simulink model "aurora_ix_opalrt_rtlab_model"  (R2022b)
settings: Solver=ode3  StartTime=0.0  StopTime=inf  FixedStep=Ts  RelTol=1e-3
PostLoadFcn:
  | aurora_ix_opalrt_rtlab_param;
InitFcn:
  | aurora_ix_opalrt_rtlab_param;
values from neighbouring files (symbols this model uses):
  Ts = 20e-6    (= 2e-05)    [aurora_ix_opalrt_rtlab_param.m]
undefined symbols (not defined in the file or in its folder): af15, arm1_g1, aurora_ix_opalrt_rtlab, aurora_ix_opalrt_rtlab_ehs, aurora_ix_opalrt_rtlab_model, aurora_ix_opalrt_rtlab_param, Boost2lvl_SFun, boost_I, boost_V, C, c62c8459, DB, EFPGASIMConfig, eHSBuildReport, eHSx64_Gen4_Machines_IOConfig1, EX, fault_sw, LABv2024, logs, matlab, Min, models, ns, OPAL, RT, Step, TE0741_3, Time, Users, v1, vin, vsrc1, vsrc2, vsrc3
libraries: rtlab x5, opal_lib x3, rtio_opalrt_common x3, monitoringUserLib x1, ehsSchematicEditorSourceLib x1

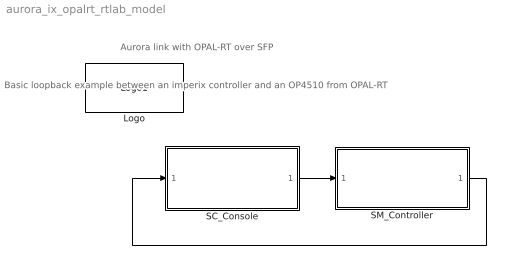
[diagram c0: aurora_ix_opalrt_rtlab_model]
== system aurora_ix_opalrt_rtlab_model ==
  note: Aurora link with OPAL-RT over SFP
  note: Basic loopback example between an imperix controller and an OP4510 from OPAL-RT
  Logo : opal_lib/Logo1  vide=[]
  SC_Console : Subsystem
  SM_Controller : Subsystem
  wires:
  SC_Console/1(to_eHS) -> SM_Controller/1(to_eHS)
  SM_Controller/1(from_eHS) -> SC_Console/1(from_eHS)

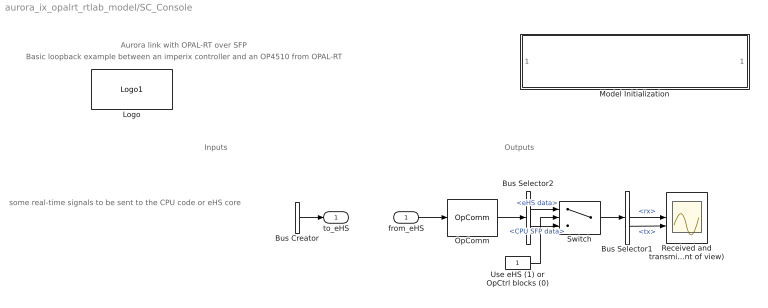
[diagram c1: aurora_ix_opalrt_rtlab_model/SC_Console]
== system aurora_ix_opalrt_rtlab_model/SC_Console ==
  note: some real-time signals to be sent to the CPU code or eHS core
  note: Inputs
  note: Outputs
  note: Aurora link with OPAL-RT over SFP
  note: Basic loopback example between an imperix controller and an OP4510 from OPAL-RT
  from_eHS : Inport  OutDataTypeStr=double
  Bus Creator : BusCreator  Inputs=2
  Bus Selector1 : BusSelector  OutputSignals=rx,tx
  Bus Selector2 : BusSelector  OutputSignals=eHS data,CPU SFP data
  Logo : opal_lib/Logo1  vide=[]
  Model Initialization : Subsystem  mask(Model Functions){InitFcnX=aurora_ix_opalrt_rtlab_param;, prel=off, posl=on, inif=on, strf=off}
      mask prompts: InitFcnX "Initialisation"; prel "Preload Function"; posl "PostLoad Function"; inif "InitFcn"; strf "StartFcn"
      mask init:
      | currentBlock = gcb;
      | root = bdroot(currentBlock);
      | 
      | if ~strcmp(get_param(root,'BlockDiagramType'),'library')
      |     if prel==1
      |         set_param(root, 'PreLoadFcn', InitFcnX);
      |     else
      |         set_param(root, 'PreLoadFcn', '');
      |     end
      |     if inif==1
      |         set_param(root, 'InitFcn', InitFcnX);
      |     else
      |         set_param(root, 'InitFcn', '');
      |     end
      |     if strf==1
      |         set_param(root, 'StartFcn', InitFcnX);
      |     else
      |         set_param(root, 'StartFcn', '');
      |     end
      |     if posl==1
      |         set_param(root, 'PostLoadFcn', InitFcnX);
      |     else
      |         set_param(root, 'PostLoadFcn', '');
      |     end
      | end
      | 
      | pos = get_param(currentBlock, 'Position');
      | width = pos(3) - pos(1); height = pos(4) - pos(2);
      | txt = [ upper(root) '\n' '- InitFcn. . . . . '  get_param(root, 'InitFcn') ];
  OpComm : rtlab/OpComm  nbport=1  groupe_acq=1  subsys_rate=0  st=0  Synchronization=off  Interpolation=off  Threshold=1.0  Missed_Data=off  Sim_Time=off  Samples=off  dynSigOut=off  from_console=0  warning_done=off  writeOpCommFile=off
  Received and transmitted signals (OP4510 point of view) : Scope  NumInputPorts=2
  Switch : Switch  Criteria=u2 ~= 0  Threshold=2
  Use eHS (1) or OpCtrl blocks (0) : Constant
  to_eHS : Outport  VectorParamsAs1DForOutWhenUnconnected=off
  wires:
  from_eHS/1 -> OpComm/1
  Bus Creator/1 -> to_eHS/1
  OpComm/1 -> Bus Selector2/1
  Bus Selector1/1 -> Received and transmitted signals (OP4510 point of view)/1  "<rx>"
  Bus Selector1/2 -> Received and transmitted signals (OP4510 point of view)/2  "<tx>"
  ? -> Bus Creator/1
  ? -> Bus Creator/2
  Bus Selector2/1 -> Switch/1  "<eHS data>"
  Bus Selector2/2 -> Switch/3  "<CPU SFP data>"
  Switch/1 -> Bus Selector1/1
  Use eHS (1) or OpCtrl blocks (0)/1 -> Switch/2

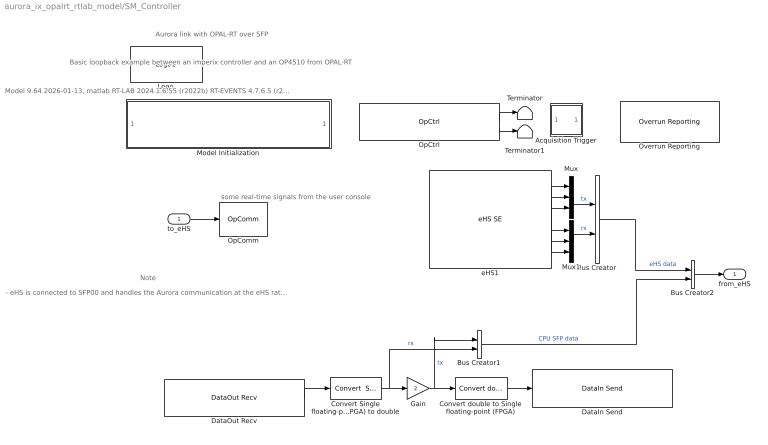
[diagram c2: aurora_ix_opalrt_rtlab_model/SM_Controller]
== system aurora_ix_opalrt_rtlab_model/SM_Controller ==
  note: Note
  note: - eHS is connected to SFP00 and handles the Aurora communication at the eHS rate - OpCtrl blocks are connected to SFP02 and handle the Aurora communication at the CPU rate
  note: Model 9.64 2026-01-13, matlab RT-LAB 2024.1.6.55 (r2022b) RT-EVENTS 4.7.6.5 (r2022b.x) eFPGAsim () &copy; 2026 Opal-RT Technologies Inc.
  note: Aurora link with OPAL-RT over SFP
  note: Basic loopback example between an imperix controller and an OP4510 from OPAL-RT
  note: some real-time signals from the user console
  to_eHS : Inport
  Acquisition Trigger : Subsystem
  Bus Creator : BusCreator  Inputs=2
  Bus Creator1 : BusCreator  Inputs=2
  Bus Creator2 : BusCreator  Inputs=2
  Convert Single floating-point (FPGA) to double : rtlab/Miscellaneous/Convert  Single floating-point (FPGA)  to double
  Convert double to Single floating-point (FPGA) : rtlab/Miscellaneous/Convert double to  Single floating-point (FPGA)
  DataIn Send : rtio_opalrt_common/DataIn Send  CtrlName='OpCtrl'  FcnNos=37  width=3  portType=uint32  checkVersion=off  expectedId=0  expectedVersion=0  opComp=>=
  DataOut Recv : rtio_opalrt_common/DataOut Recv  CtrlName='OpCtrl'  FcnNos=15  width=3  portType=uint32  sampleTime=0  checkVersion=off  expectedId=0  expectedVersion=0  opComp=>=
  Gain : Gain  Gain=2
  Logo : opal_lib/Logo1  vide=[]
  Model Initialization : Subsystem  mask(Model Functions){InitFcnX=aurora_ix_opalrt_rtlab_param;, prel=off, posl=on, inif=on, strf=off}
      mask prompts: InitFcnX "Initialisation"; prel "Preload Function"; posl "PostLoad Function"; inif "InitFcn"; strf "StartFcn"
      mask init:
      | currentBlock = gcb;
      | root = bdroot(currentBlock);
      | 
      | if ~strcmp(get_param(root,'BlockDiagramType'),'library')
      |     if prel==1
      |         set_param(root, 'PreLoadFcn', InitFcnX);
      |     else
      |         set_param(root, 'PreLoadFcn', '');
      |     end
      |     if inif==1
      |         set_param(root, 'InitFcn', InitFcnX);
      |     else
      |         set_param(root, 'InitFcn', '');
      |     end
      |     if strf==1
      |         set_param(root, 'StartFcn', InitFcnX);
      |     else
      |         set_param(root, 'StartFcn', '');
      |     end
      |     if posl==1
      |         set_param(root, 'PostLoadFcn', InitFcnX);
      |     else
      |         set_param(root, 'PostLoadFcn', '');
      |     end
      | end
      | 
      | pos = get_param(currentBlock, 'Position');
      | width = pos(3) - pos(1); height = pos(4) - pos(2);
      | txt = [ upper(root) '\n' '- InitFcn. . . . . '  get_param(root, 'InitFcn') ];
  Mux : Mux  Inputs=3
  Mux1 : Mux  Inputs=3
  OpComm : rtlab/OpComm  nbport=1  groupe_acq=1  subsys_rate=0  st=0  Synchronization=on  Interpolation=on  Threshold=1.0  Missed_Data=off  Sim_Time=off  Samples=off  dynSigOut=off  from_console=1  warning_done=off  writeOpCommFile=off
  OpCtrl : rtio_opalrt_common/OpCtrl  CtrlName='OpCtrl'  boardid=0  BitstreamFilename=TE0741_3-EX-0001-3_11_2_12-eHSx64_Gen4_Machines_IOConfig1-DB-4A.bin  numconfig=-1  mode=Master  externalClock=off  decimRtsi=0  calibIO=off  SampleTime=0  loadinport=-1  BoardType=TE0741  SecondaryPresent=off  sync_type=Audio  scope_enable=off  fsdFileName=TE0741_3-EX-0001-3_11_2_12-eHSx64_Gen4_Machines_IOConfig1-DB-4A.fsd  mismatch_disable=on
  Overrun Reporting : monitoringUserLib/Overrun Reporting  acquisitionGroup=26  simTimeSeconds=2  startTimeSeconds=0.5  timeStep=Ts
  Terminator : Terminator
  Terminator1 : Terminator
  eHS1 : ehsSchematicEditorSourceLib/eHS SE  modelName=Boost2lvl_SFun - v1  modelUuid=c62c8459-3f79-48c0-af15-759a73c628dc  modelDisplayName=Boost2lvl_SFun  lastLoadedModelText=Circuit loaded on 09-Oct-2024 14:20:43  lastLoadedModelName=Boost2lvl_SFun - v1  lastLoadedModelUuid=c62c8459-3f79-48c0-af15-759a73c628dc  lastLoadedModelDisplayName=Boost2lvl_SFun - v1  triggerUpdate=on  timeStepInfo=Time Step: 230 ns (Min: 230 ns)  inputPins=arm1_g1,fault_sw,vin,vsrc1,vsrc2,vsrc3  outputPins=2Lvl_Ia,2Lvl_Ib,2Lvl_Ic,2Lvl_Va,2Lvl_Vb,2Lvl_Vc,boost_I,boost_V  loadPassed=1  firmwareName=TE0741_3-EX-0001-3_11_2_12-eHSx64_Gen4_Machines_IOConfig1-DB-4A.bin  driverType=SFUN  ehsEffectiveLicense=x128  migrated=on  opCtrlName='OpCtrl'  autoConfigureFirmware=on  ehsFileName=aurora_ix_opalrt_rtlab_ehs.ehs3  buildReportFile=C:\Users\matlab\OPAL-RT\RT-LABv2024.1_Workspace\aurora_ix_opalrt_rtlab\models\aurora_ix_opalrt_rtlab_model\EFPGASIMConfig\logs\aurora_ix_opalrt_rtlab_ehs\logs\eHSBuildReport.txt  displayBlockInfos=|
      | x32
      | Time Step: 205 ns (Min: 205 ns)
  from_eHS : Outport  VectorParamsAs1DForOutWhenUnconnected=off
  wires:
  to_eHS/1 -> OpComm/1
  OpComm/1 -> ?
  Bus Creator/1 -> Bus Creator2/1  "eHS data"
  OpCtrl/1 -> Terminator/1
  OpCtrl/2 -> Terminator1/1
  eHS1/2 -> Mux/2
  eHS1/3 -> Mux/3
  eHS1/5 -> Mux1/2
  eHS1/6 -> Mux1/3
  eHS1/4 -> Mux1/1
  Mux1/1 -> Bus Creator/2  "rx"
  DataOut Recv/1 -> Convert Single floating-point (FPGA) to double/1
  Gain/1 -> Bus Creator1/1, Convert double to Single floating-point (FPGA)/1  "tx"
  Convert Single floating-point (FPGA) to double/1 -> Bus Creator1/2, Gain/1  "rx"
  Convert double to Single floating-point (FPGA)/1 -> DataIn Send/1
  Bus Creator1/1 -> Bus Creator2/2  "CPU SFP data"
  Bus Creator2/1 -> from_eHS/1
  eHS1/1 -> Mux/1
  Mux/1 -> Bus Creator/1  "tx"

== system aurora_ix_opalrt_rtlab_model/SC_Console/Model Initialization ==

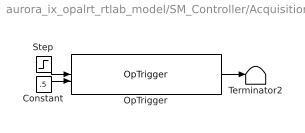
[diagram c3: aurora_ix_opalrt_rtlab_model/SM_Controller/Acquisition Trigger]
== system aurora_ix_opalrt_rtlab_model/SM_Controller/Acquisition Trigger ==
  Constant : Constant  Value=.5
  OpTrigger : rtlab/DataLogging/OpTrigger  Trig_Type=TRIGGER SIGNAL >= TRIGGER LEVEL  Trig_Offset=0  Acq_Group=1
  Step : Step  Time=0.5  SampleTime=Ts
  Terminator2 : Terminator
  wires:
  Constant/1 -> OpTrigger/2
  Step/1 -> OpTrigger/1
  OpTrigger/1 -> Terminator2/1

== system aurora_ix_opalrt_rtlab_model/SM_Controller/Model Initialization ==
